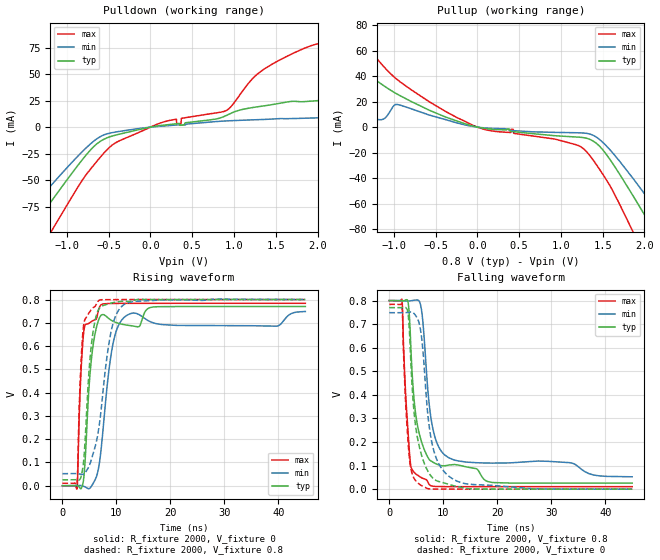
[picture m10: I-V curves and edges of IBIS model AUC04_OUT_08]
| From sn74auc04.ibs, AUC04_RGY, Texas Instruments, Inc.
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[Model]   AUC04_OUT_08
Model_type  Output
Vref =   0
Rref =   2000
Cref =   15p
Vmeas =   0.4
| variable   typ   min   max
C_comp   3.5pF   NA   NA
| C_pullup   5.60pF   2.30pF   8.10pF
| C_pulldown   6.44pF   5.86pF   6.78pF
[Temperature Range]   40   100   -40
| Ambient temperature   25   85   -40
[Voltage range]   0.8   0.8   0.8
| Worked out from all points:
|   slope of the pulldown table from 0 to 0.12 V, typ, clamps not added: 76.3 ohm
|   slope of the pullup table from 0 to 0.12 V, typ, clamps not added: 91.4 ohm
|   rising waveform, R_fixture 2000, V_fixture 0: 20-80 % time 1.45ns typ, 2.14ns min, 863ps max; typ from 0 V to 0.77 V
|   falling waveform, R_fixture 2000, V_fixture 0.8: 20-80 % time 2.36ns typ, 2.3ns min, 1.11ns max; typ from 0.8 V to 0.026 V
|   rising waveform, R_fixture 2000, V_fixture 0.8: 20-80 % time 1.42ns typ, 2.51ns min, 805ps max; typ from 0.025 V to 0.8 V
|   falling waveform, R_fixture 2000, V_fixture 0: 20-80 % time 2ns typ, 2.23ns min, 1.06ns max; typ from 0.77 V to 0 V
[Pulldown]
| AUC04_OUT_08
|   Voltage   I(typ)   I(min)   I(max)
-3.6V     -337.3mA   -282.2mA   -412.4mA
-1.79V    -136.5mA   -110mA     -177.8mA
-1.39V    -92.23mA   -73.02mA   -125.2mA
-1.17V    -68.14mA   -53.2mA    -96.14mA
-685mV    -18.8mA    -13.58mA   -36.41mA
-430mV    -7.788mA   -4.787mA   -15.34mA
165mV     1.975mA    1.123mA    5.083mA
905mV     10.9mA     5.849mA    15.59mA
1.32V     19.64mA    7.147mA    52.55mA
2.005V    25.03mA    8.767mA    78.7mA
3.335V    32.94mA    11.65mA    90.33mA
7.2V      56.65mA    21.1mA     140.7mA
[Pullup]
| AUC04_OUT_08
|   Voltage   I(typ)   I(min)   I(max)
-3.6V     112.9mA    15.55mA    196mA
-2.685V   76.06mA    17.84mA    164mA
-1.875V   36.81mA    19.48mA    111.1mA
-1.505V   32.64mA    11.52mA    78.71mA
-1.285V   39.44mA    7.211mA    60.37mA
-960mV    25.93mA    17.8mA     37.34mA
-245mV    4.855mA    3.296mA    7.535mA
1.26V     -8.135mA   -4.57mA    -16.37mA
1.87V     -54.47mA   -40.74mA   -82.92mA
2.04V     -72.97mA   -55.67mA   -106mA
2.465V    -120.2mA   -94.46mA   -163.4mA
7.2V      -650.8mA   -549.9mA   -789.4mA
[Ramp]
| AUC04_OUT_08
| variable   typ   min   max
dV/dt_r   0.47/1.46E-09   0.46/2.17E-09   0.48/8.66E-10
dV/dt_f   0.47/2.35E-09   0.45/2.29E-09   0.48/1.11E-09
R_load = 2000
[Rising Waveform]
| AUC04_OUT_08
R_fixture =   2000
C_fixture =   0
L_fixture =   0
V_fixture =   0
V_fixture_min = 0
V_fixture_max = 0
|   Time   V(typ)   V(min)   V(max)
0s        10.85nV    62.38nV    582.1pV
2.73ns    769.1uV    1.107mV    -9.049mV
3.25ns    -10.38mV   1.016mV    389.4mV
3.785ns   8.327mV    -1.054mV   619.2mV
5.385ns   547.6mV    -1.606mV   705.5mV
7.16ns    732.1mV    154.9mV    777.4mV
9.275ns   707.8mV    599.1mV    783.1mV
11.82ns   690.4mV    730.5mV    783.5mV
16.84ns   768mV      699.6mV    783.6mV
45ns      770mV      748.7mV    783.7mV
[Falling Waveform]
| AUC04_OUT_08
R_fixture =   2000
C_fixture =   0
L_fixture =   0
V_fixture =   0.8
V_fixture_min = 0.8
V_fixture_max = 0.8
|   Time   V(typ)   V(min)   V(max)
0s        800mV      800mV      800mV
2.34ns    799.2mV    799.8mV    802.2mV
3.455ns   796.1mV    798.3mV    249.1mV
3.975ns   611.2mV    799.1mV    100.3mV
4.56ns    387.9mV    801.4mV    72.4mV
5.66ns    226mV      791.9mV    52.84mV
7.545ns   122.3mV    330.1mV    16.53mV
9.12ns    103.1mV    180.8mV    11.18mV
12.05ns   104.6mV    123.4mV    10.78mV
45ns      25.56mV    52.48mV    10.62mV
[Rising Waveform]
| AUC04_OUT_08
R_fixture =   2000
C_fixture =   0
L_fixture =   0
V_fixture =   0.8
V_fixture_min = 0.8
V_fixture_max = 0.8
|   Time   V(typ)   V(min)   V(max)
0s        25.46mV    51.93mV    10.6mV
2.705ns   25.49mV    52.15mV    11.42mV
3.165ns   25.9mV     50.66mV    373.4mV
3.545ns   47.75mV    49.12mV    573.7mV
4.035ns   135.8mV    51.25mV    703.4mV
5.29ns    589.4mV    107.1mV    754.7mV
6.745ns   758.8mV    248.3mV    795.5mV
8.995ns   784.4mV    660.3mV    799.5mV
11.47ns   792.3mV    779.3mV    799.7mV
45ns      800mV      800.1mV    800mV
[Falling Waveform]
| AUC04_OUT_08
R_fixture =   2000
C_fixture =   0
L_fixture =   0
V_fixture =   0
V_fixture_min = 0
V_fixture_max = 0
|   Time   V(typ)   V(min)   V(max)
0s        770mV      748.6mV    783.8mV
2.325ns   769.5mV    748.5mV    783.3mV
2.905ns   771.4mV    748.5mV    424.4mV
3.4ns     755.1mV    749.7mV    226.5mV
3.885ns   597mV      751.2mV    98.89mV
4.52ns    343.5mV    746.4mV    48.75mV
5.62ns    174.3mV    695.6mV    20.19mV
7.835ns   52.62mV    203.6mV    803.7uV
11.2ns    18.91mV    51.97mV    180.7uV
45ns      70.06uV    30.7uV     20.39uV
